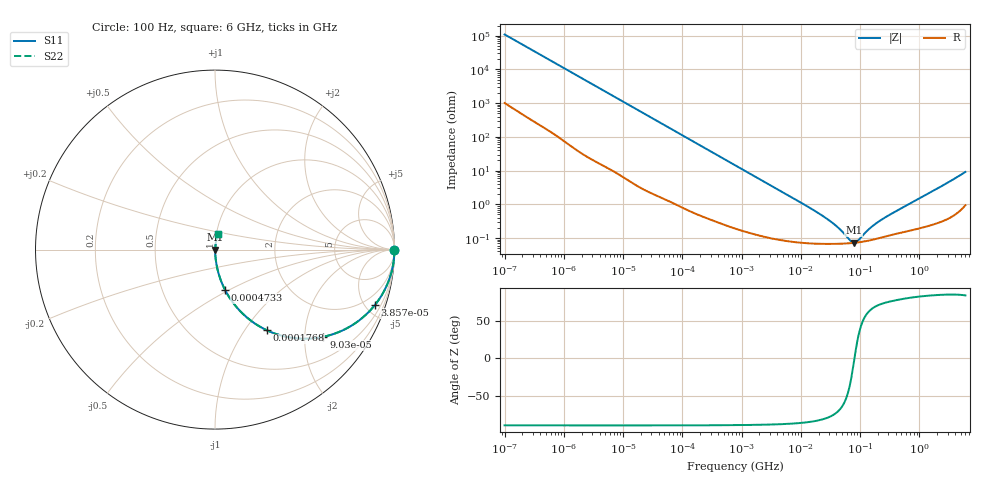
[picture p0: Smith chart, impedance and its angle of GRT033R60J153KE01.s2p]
!Murata Part Number: GRT033R60J153KE01
!These Parameters are Measured in Series Mode Connection
!Data Generated on Jun 19, 2026
!  o--ll--o
!Port1  Port2
!  o------o
!Operation Temp=25[degC], DC Bias Voltage=0[V]
!Freq. Start=100[Hz] Stop=6[GHz] 401[Steps]
# Hz S RI R 50
!Freq.(Hz) S11(Real) S11(Imag) S21(Real) S21(Imag) S12(Real) S12(Imag) S22(Real) S22(Imag)
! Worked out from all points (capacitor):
!   401 points, 100 Hz to 6 GHz, reference 50 ohm
!   read as one part in series: C = 14.6 nF near 109 Hz
!   lowest |Z| = 72.4 mohm at 77.97 MHz (marker M1)
!   series resonance near 80.47 MHz, so ESL is about 270 pH
!   S11 on the Smith chart (normalised r, x): 100 Hz: open; 38.57 kHz: 1.03, -5.77; 90.3 kHz: 1.02, -2.47; 176.8 kHz: 1.01, -1.27; 473.3 kHz: 1.01, -0.48; 6 GHz: 1.02, +0.18
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100  1 -0.000921  9.4e-06 0.000921  9.4e-06 0.000921  1 -0.000921
2008  0.9996 -0.0182  0.000438 0.0182  0.000438 0.0182  0.9996 -0.0182
11514  0.9888 -0.1026  0.0112 0.1026  0.0112 0.1026  0.9888 -0.1026
38569  0.8913 -0.3082  0.1087 0.3082  0.1087 0.3082  0.8913 -0.3082
40335  0.8824 -0.3191  0.1176 0.3191  0.1176 0.3191  0.8824 -0.3191
60352  0.7719 -0.4163  0.2281 0.4163  0.2281 0.4163  0.7719 -0.4163
90302  0.604 -0.4856  0.396 0.4856  0.396 0.4856  0.604 -0.4856
176758  0.2879 -0.4488  0.7121 0.4488  0.7121 0.4488  0.2879 -0.4488
276587  0.1436 -0.3461  0.8564 0.3461  0.8564 0.3461  0.1436 -0.3461
473344  0.0557 -0.2239  0.9443 0.2239  0.9443 0.2239  0.0557 -0.2239
774597  0.0226 -0.1421  0.9774 0.1421  0.9774 0.1421  0.0226 -0.1421
2481164  0.00316 -0.0456  0.9968 0.0456  0.9968 0.0456  0.00316 -0.0456
1.555665e7  0.000738 -0.00709  0.9993 0.00709  0.9993 0.00709  0.000738 -0.00709
3.482834e7  0.000678 -0.00267  0.9993 0.00267  0.9993 0.00267  0.000678 -0.00267
4.764863e7  0.000682 -0.00156  0.9993 0.00156  0.9993 0.00156  0.000682 -0.00156
6.817316e7  0.000704 -0.000471  0.9993 0.000471  0.9993 0.000471  0.000704 -0.000471
7.797396e7  0.000718 -8.83e-05  0.9993 8.83e-05  0.9993 8.83e-05  0.000718 -8.83e-05
8.918374e7  0.000737 0.00029  0.9993 -0.00029  0.9993 -0.00029  0.000737 0.00029
1.745687e8  0.000922 0.00232  0.9991 -0.00232  0.9991 -0.00232  0.000922 0.00232
3.124326e8  0.00121 0.00469  0.9988 -0.00469  0.9988 -0.00469  0.00121 0.00469
1.95892e9  0.00351 0.0283  0.9965 -0.0283  0.9965 -0.0283  0.00351 0.0283
6e9  0.0173 0.0885  0.9827 -0.0885  0.9827 -0.0885  0.0173 0.0885
